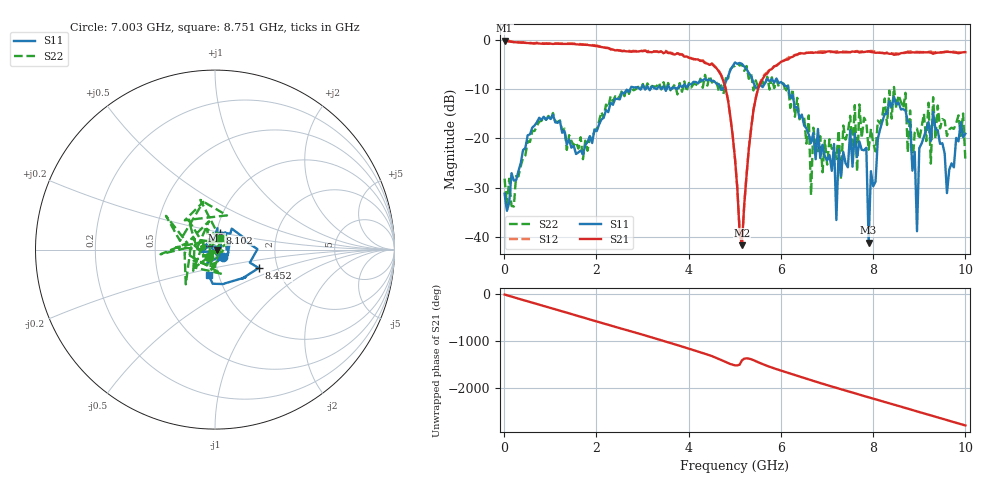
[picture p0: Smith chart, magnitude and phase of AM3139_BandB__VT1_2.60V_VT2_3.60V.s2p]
! Date/Time: Tue, Nov 13, 2018 5:00 PM
! Network Analyzer: Agilent Technologies E8364B Rev: A.07.50.67
! Sweep from 0.010 to 10.000 GHz, 201 Points, Sweep Type: LIN
! Power Supply: 2.601 V, 0.000 A
# Hz S DB R 50
!freq MagS11 AngS11 MagS21 AngS21 MagS12 AngS12 MagS22 AngS22
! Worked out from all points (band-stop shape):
!   201 points, 10 MHz to 10 GHz, reference 50 ohm
!   highest |S21| = -0.17 dB at 10 MHz (marker M1); lowest = -41.7 dB at 5.155 GHz (marker M2)
!   |S21| within 3 dB of the highest: start of sweep to 3.873 GHz; 6.303 GHz to end of sweep
!   lowest |S11| = -41.2 dB at 7.902 GHz (marker M3), VSWR 1.02, Z = 50.9 - j0.19 ohm
!   |S11| at or under -10 dB: start of sweep to 2.736 GHz; 2.942 GHz to 2.964 GHz (22.68 MHz wide, 0.768 % of centre); 6.166 GHz to end of sweep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
!   |S22| runs from -33.9 to -4.7 dB; largest |S21 - S12| = 0.033
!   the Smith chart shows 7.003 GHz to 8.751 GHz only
!   S11 on the Smith chart (normalised r, x): 7.003 GHz: 1.08, -0.09; 8.102 GHz: 1.04, +0.20; 8.452 GHz: 1.60, -0.35; 8.751 GHz: 0.90, -0.26
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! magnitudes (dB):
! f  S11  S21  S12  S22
! 10 MHz  -31.3  -0.2  -0.2  -28.2
! 1.708 GHz  -23.3  -1.0  -1.0  -24.3
! 3.357 GHz  -9.4  -2.5  -2.5  -8.7
! 4.655 GHz  -9.0  -6.5  -6.3  -10.5
! 5.005 GHz  -4.6  -24.1  -24.1  -5.3
! 5.155 GHz  -4.9  -41.7  -41.9  -5.0
! 5.554 GHz  -9.2  -8.8  -8.6  -9.7
! 6.603 GHz  -19.2  -2.6  -2.7  -15.3
! 6.653 GHz  -21.0  -2.6  -2.6  -31.5
! 6.703 GHz  -19.0  -2.7  -2.6  -17.9
! 7.003 GHz  -24.5  -2.4  -2.5  -25.3
! 7.852 GHz  -21.9  -2.4  -2.5  -16.7
! 7.902 GHz  -41.2  -2.4  -2.4  -22.3
! 8.102 GHz  -20.1  -2.6  -2.6  -16.4
! 8.352 GHz  -12.5  -2.9  -2.8  -10.3
! 8.452 GHz  -11.6  -3.1  -2.9  -9.6
! 8.751 GHz  -16.6  -2.6  -2.4  -22.9
! 8.951 GHz  -38.9  -2.6  -2.5  -18.0
! 9.001 GHz  -22.0  -2.6  -2.5  -20.2
! 9.301 GHz  -14.7  -2.9  -2.6  -11.7
! 9.6 GHz  -31.1  -2.5  -2.4  -19.5
! 10 GHz  -19.1  -2.5  -2.5  -24.6
